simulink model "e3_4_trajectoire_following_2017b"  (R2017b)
settings: Solver=FixedStepAuto  StartTime=0.0  StopTime=150  FixedStep=sampleTime  RelTol=1e-3  EnableMultiTasking=on
InitFcn:
  | start;
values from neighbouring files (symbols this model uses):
  k_d_x = 1.65    [start.m]    (also in StartSimulation.m = 1.5; startSimulation.m = 1.5)
  k_d_y = 1.52    [start.m]    (also in StartSimulation.m = 1.5; startSimulation.m = 1.5)
  k_d_yaw = 1    [start.m]    (also in StartSimulation.m; startSimulation.m)
  k_d_z = 0.5    [start.m]    (also in StartSimulation.m; startSimulation.m)
  k_i_x = 0.9    [start.m]    (also in StartSimulation.m = 0.01; startSimulation.m = 0.01)
  k_i_y = 0.91    [start.m]    (also in StartSimulation.m = 0.01; startSimulation.m = 0.01)
  k_i_yaw = 0.01    [start.m]    (also in StartSimulation.m; startSimulation.m)
  k_i_z = 0.01    [start.m]    (also in StartSimulation.m; startSimulation.m)
  k_p_x = 1.9    [start.m]    (also in StartSimulation.m = 1.2; startSimulation.m = 1.2)
  k_p_y = 1.9    [start.m]    (also in StartSimulation.m = 1.5; startSimulation.m = 1.5)
  k_p_yaw = 2    [start.m]    (also in StartSimulation.m; startSimulation.m)
  k_p_z = 2    [start.m]    (also in StartSimulation.m; startSimulation.m)
  saturation_psi = 2    [start.m]    (also in StartSimulation.m; startSimulation.m)
  saturation_x = 2    [start.m]    (also in StartSimulation.m; startSimulation.m)
  saturation_y = 2    [start.m]    (also in StartSimulation.m; startSimulation.m)
  saturation_z = 2    [start.m]    (also in StartSimulation.m; startSimulation.m)
libraries: simulink x36, aerolibanimutils x1

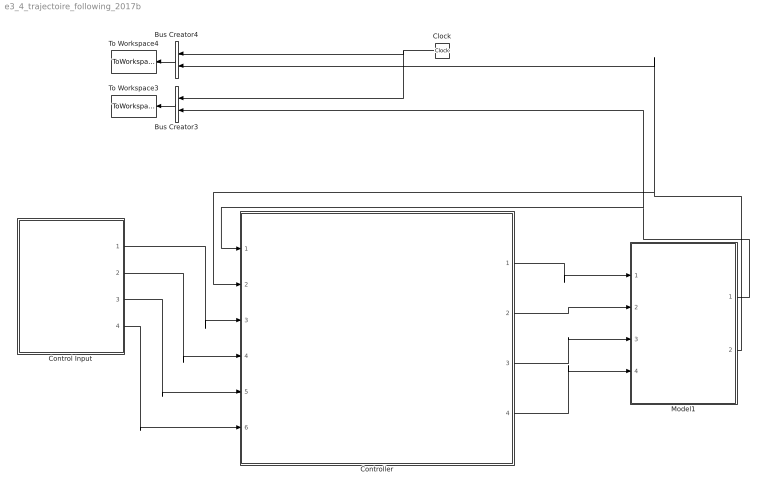
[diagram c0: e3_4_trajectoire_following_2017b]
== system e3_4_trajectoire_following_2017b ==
  Bus Creator3 : BusCreator  Inputs=2
  Bus Creator4 : BusCreator  Inputs=2
  Clock : Clock
  Control Input : Subsystem
  Controller : Subsystem
  Model1 : Subsystem
  To Workspace3 : ToWorkspace  VariableName=r1_pos_array1  SampleTime=-1
  To Workspace4 : ToWorkspace  VariableName=r1_vel_array1  SampleTime=-1
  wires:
  Controller/2(Controller Output Y) -> Model1/2(uy)
  Controller/3(Controller Output H) -> Model1/3(uz)
  Controller/4(Controller Output Psi) -> Model1/4(upsi)
  Model1/2(Output Velocity1) -> Bus Creator4/2, Controller/2(Feedback Velocity)
  Model1/1(Output Postion1) -> Bus Creator3/2, Controller/1(Feedback Position)
  Bus Creator3/1 -> To Workspace3/1
  Clock/1 -> Bus Creator3/1, Bus Creator4/1
  Bus Creator4/1 -> To Workspace4/1
  Control Input/2(uy) -> Controller/4(Control input Y)
  Control Input/1(ux) -> Controller/3(Control input X)
  Control Input/3(uz) -> Controller/5(Control input H)
  Control Input/4(upsi) -> Controller/6(Control input Psi)
  Controller/1(Controller Output X) -> Model1/1(ux)

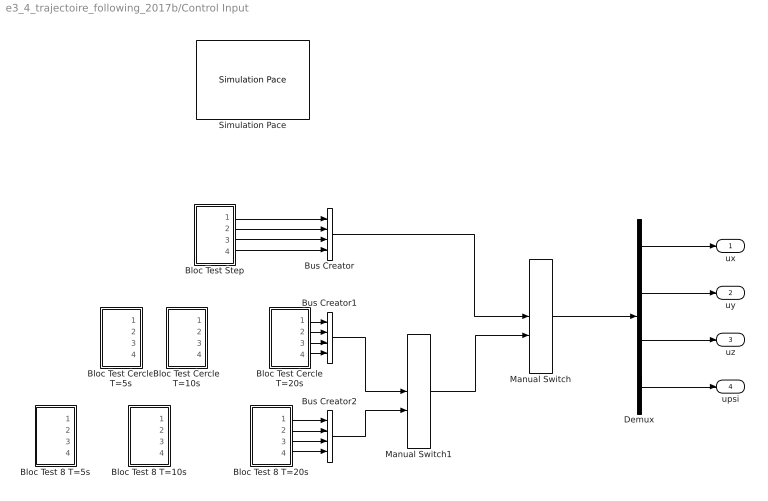
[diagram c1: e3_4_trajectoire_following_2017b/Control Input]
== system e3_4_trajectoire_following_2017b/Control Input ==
  Bloc Test 8 T=10s : Subsystem
  Bloc Test 8 T=20s : Subsystem
  Bloc Test 8 T=5s : Subsystem
  Bloc Test Cercle T=10s : Subsystem
  Bloc Test Cercle T=20s : Subsystem
  Bloc Test Cercle T=5s : Subsystem
  Bloc Test Step : Subsystem
  Bus Creator : BusCreator  Inputs=4
  Bus Creator1 : BusCreator  Inputs=4
  Bus Creator2 : BusCreator  Inputs=4
  Demux : Demux
  Manual Switch : ManualSwitch  CurrentSetting=0
  Manual Switch1 : ManualSwitch
  Simulation Pace : aerolibanimutils/Simulation Pace  SimulationPace=100  SleepMode=MATLAB Thread  OutputPaceError=off  SampleTime=-1
  ux : Outport  VectorParamsAs1DForOutWhenUnconnected=off
  uy : Outport  Port=2  VectorParamsAs1DForOutWhenUnconnected=off
  uz : Outport  Port=3  VectorParamsAs1DForOutWhenUnconnected=off
  upsi : Outport  Port=4  VectorParamsAs1DForOutWhenUnconnected=off
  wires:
  Demux/2 -> uy/1
  Demux/1 -> ux/1
  Bloc Test Step/2(uy) -> Bus Creator/2
  Demux/3 -> uz/1
  Demux/4 -> upsi/1
  Bloc Test Step/4(upsi) -> Bus Creator/4
  Bloc Test Step/3(uz) -> Bus Creator/3
  Bloc Test Step/1(ux) -> Bus Creator/1
  Bus Creator/1 -> Manual Switch/1
  Bus Creator1/1 -> Manual Switch1/1
  Bus Creator2/1 -> Manual Switch1/2
  Manual Switch/1 -> Demux/1
  Manual Switch1/1 -> Manual Switch/2
  Bloc Test 8 T=20s/1(ux) -> Bus Creator2/1
  Bloc Test 8 T=20s/2(uy) -> Bus Creator2/2
  Bloc Test 8 T=20s/3(uz) -> Bus Creator2/3
  Bloc Test 8 T=20s/4(upsi) -> Bus Creator2/4
  Bloc Test Cercle T=20s/1(ux) -> Bus Creator1/1
  Bloc Test Cercle T=20s/2(uy) -> Bus Creator1/2
  Bloc Test Cercle T=20s/3(uz) -> Bus Creator1/3
  Bloc Test Cercle T=20s/4(upsi) -> Bus Creator1/4

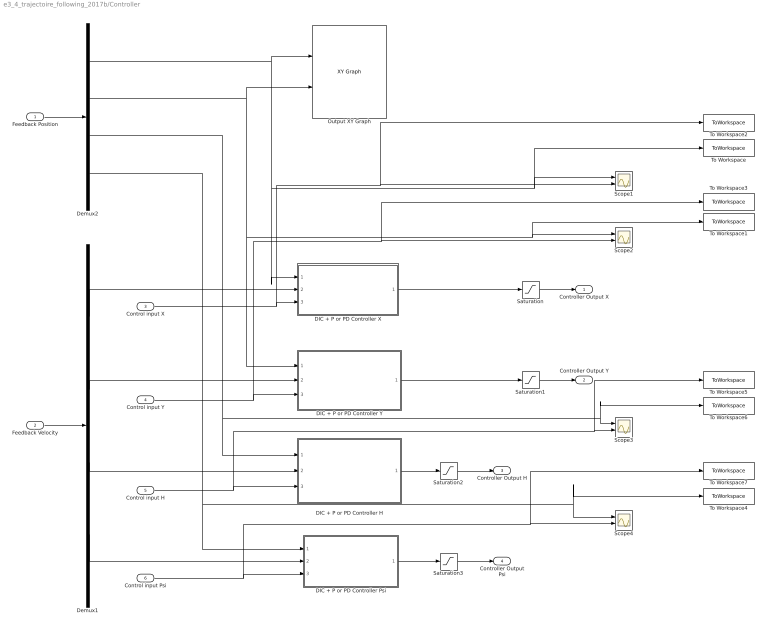
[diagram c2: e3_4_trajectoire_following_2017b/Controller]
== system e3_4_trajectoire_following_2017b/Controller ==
  Feedback Position : Inport
  Feedback Velocity : Inport  Port=2
  Control input X : Inport  Port=3
  Control input Y : Inport  Port=4
  Control input H : Inport  Port=5
  Control input Psi : Inport  Port=6
  DIC + P or PD Controller H : Subsystem
  DIC + P or PD Controller Psi : Subsystem
  DIC + P or PD Controller X : Subsystem
  DIC + P or PD Controller Y : Subsystem
  Demux1 : Demux
  Demux2 : Demux
  Output XY Graph : simulink/Sinks/XY Graph  xmin=-1  xmax=1  ymin=-1  ymax=1  st=-1
  Saturation : Saturate  UpperLimit=saturation_x  LowerLimit=-saturation_x
  Saturation1 : Saturate  UpperLimit=saturation_y  LowerLimit=-saturation_y
  Saturation2 : Saturate  UpperLimit=saturation_z  LowerLimit=-saturation_z
  Saturation3 : Saturate  UpperLimit=saturation_psi  LowerLimit=-saturation_psi
  Scope{1..4} (4 alike) : Scope  NumInputPorts=2
  To Workspace : ToWorkspace  VariableName=N4_Step1_Out_X  SampleTime=-1
  To Workspace1 : ToWorkspace  VariableName=N4_Step1_Out_Y  SampleTime=-1
  To Workspace2 : ToWorkspace  VariableName=N4_Step1_In_X  SampleTime=-1
  To Workspace3 : ToWorkspace  VariableName=N4_Step1_In_Y  SampleTime=-1
  To Workspace4 : ToWorkspace  VariableName=N4_Step1_Out_Psi  SampleTime=-1
  To Workspace5 : ToWorkspace  VariableName=N4_Step1_In_H  SampleTime=-1
  To Workspace6 : ToWorkspace  VariableName=N4_Step1_Out_H  SampleTime=-1
  To Workspace7 : ToWorkspace  VariableName=N4_Step1_In_Psi  SampleTime=-1
  Controller Output X : Outport  VectorParamsAs1DForOutWhenUnconnected=off
  Controller Output Y : Outport  Port=2  VectorParamsAs1DForOutWhenUnconnected=off
  Controller Output H : Outport  Port=3  VectorParamsAs1DForOutWhenUnconnected=off
  Controller Output Psi : Outport  Port=4  VectorParamsAs1DForOutWhenUnconnected=off
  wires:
  Feedback Position/1 -> Demux2/1
  Feedback Velocity/1 -> Demux1/1
  Demux1/2 -> DIC + P or PD Controller Y/2(Feedback Velocity Y)
  Demux2/3 -> Scope3/1, To Workspace6/1, DIC + P or PD Controller H/1(Feedback Position H)
  Demux1/1 -> DIC + P or PD Controller X/2(Feedback Velocity X)
  Demux1/3 -> DIC + P or PD Controller H/2(Feedback Velocity H)
  Control input X/1 -> To Workspace2/1, Scope1/2, DIC + P or PD Controller X/3(Control Input X)
  Control input H/1 -> Scope3/2, To Workspace5/1, DIC + P or PD Controller H/3(Control Input H)
  Saturation/1 -> Controller Output X/1
  Saturation1/1 -> Controller Output Y/1
  Saturation2/1 -> Controller Output H/1
  Saturation3/1 -> Controller Output Psi/1
  Control input Y/1 -> Scope2/2, To Workspace3/1, DIC + P or PD Controller Y/3(Control Input Y)
  DIC + P or PD Controller H/1(Controller Output H) -> Saturation2/1
  DIC + P or PD Controller Psi/1(Controller Output Psi) -> Saturation3/1
  Demux2/1 -> DIC + P or PD Controller X/1(Feedback Position X), To Workspace/1, Scope1/1, Output XY Graph/1
  Demux2/2 -> Scope2/1, To Workspace1/1, DIC + P or PD Controller Y/1(Feedback Position Y), Output XY Graph/2
  Demux2/4 -> Scope4/1, To Workspace4/1, DIC + P or PD Controller Psi/1(Feedback Position Psi)
  Demux1/4 -> DIC + P or PD Controller Psi/2(Feedback Velocity Psi)
  Control input Psi/1 -> Scope4/2, To Workspace7/1, DIC + P or PD Controller Psi/3(Control input Psi)
  DIC + P or PD Controller Y/1(Controller Output Y) -> Saturation1/1
  DIC + P or PD Controller X/1(Controller Output X) -> Saturation/1

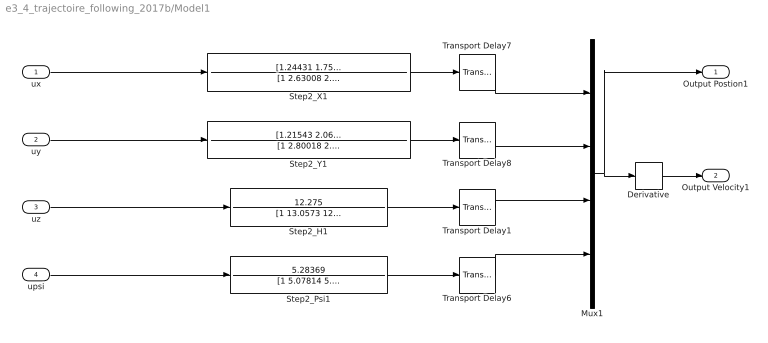
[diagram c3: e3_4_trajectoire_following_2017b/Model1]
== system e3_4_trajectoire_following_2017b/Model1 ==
  ux : Inport
  uy : Inport  Port=2
  uz : Inport  Port=3
  upsi : Inport  Port=4
  Derivative : Derivative
  Mux1 : Mux
  Step2_H1 : TransferFcn  Numerator=12.275  Denominator=[1 13.0573 12.3932]
  Step2_Psi1 : TransferFcn  Numerator=5.28369  Denominator=[1 5.07814 5.37552]
  Step2_X1 : TransferFcn  Numerator=[1.24431 1.75269]  Denominator=[1 2.63008 2.37405 1.95897]
  Step2_Y1 : TransferFcn  Numerator=[1.21543 2.06629]  Denominator=[1 2.80018 2.54762 2.23605]
  Transport Delay1 : TransportDelay  DelayTime=0.0271
  Transport Delay6 : TransportDelay  DelayTime=0.0281
  Transport Delay7 : TransportDelay  DelayTime=0.3778
  Transport Delay8 : TransportDelay  DelayTime=0.3715
  Output Postion1 : Outport
  Output Velocity1 : Outport  Port=2
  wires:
  upsi/1 -> Step2_Psi1/1
  Transport Delay8/1 -> Mux1/2
  Step2_Y1/1 -> Transport Delay8/1
  Step2_Psi1/1 -> Transport Delay6/1
  Transport Delay6/1 -> Mux1/4
  Transport Delay1/1 -> Mux1/3
  ux/1 -> Step2_X1/1
  Step2_X1/1 -> Transport Delay7/1
  Transport Delay7/1 -> Mux1/1
  Step2_H1/1 -> Transport Delay1/1
  uz/1 -> Step2_H1/1
  uy/1 -> Step2_Y1/1
  Derivative/1 -> Output Velocity1/1
  Mux1/1 -> Derivative/1, Output Postion1/1

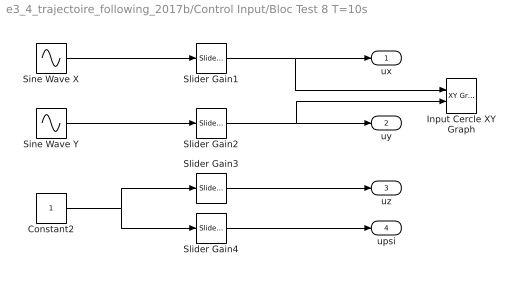
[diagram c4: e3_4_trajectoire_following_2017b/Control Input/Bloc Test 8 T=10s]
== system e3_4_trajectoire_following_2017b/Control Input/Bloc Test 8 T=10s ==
  Constant2 : Constant
  Input Cercle XY Graph : simulink/Sinks/XY Graph  xmin=-1  xmax=1  ymin=-1  ymax=1  st=-1
  Sine Wave X : Sin  Frequency=0.65  SampleTime=0
  Sine Wave Y : Sin  Frequency=1.3  SampleTime=0
  Slider Gain1 : simulink/Math Operations/Slider Gain  gain=1  low=-10  high=10
  Slider Gain2 : simulink/Math Operations/Slider Gain  gain=1  low=-10  high=10
  Slider Gain3 : simulink/Math Operations/Slider Gain  gain=1  low=-3  high=3
  Slider Gain4 : simulink/Math Operations/Slider Gain  gain=0  low=-2  high=2
  ux : Outport  VectorParamsAs1DForOutWhenUnconnected=off
  uy : Outport  Port=2  VectorParamsAs1DForOutWhenUnconnected=off
  uz : Outport  Port=3  VectorParamsAs1DForOutWhenUnconnected=off
  upsi : Outport  Port=4  VectorParamsAs1DForOutWhenUnconnected=off
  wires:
  Slider Gain2/1 -> Input Cercle XY Graph/2, uy/1
  Slider Gain3/1 -> uz/1
  Slider Gain4/1 -> upsi/1
  Slider Gain1/1 -> Input Cercle XY Graph/1, ux/1
  Constant2/1 -> Slider Gain4/1, Slider Gain3/1
  Sine Wave Y/1 -> Slider Gain2/1
  Sine Wave X/1 -> Slider Gain1/1

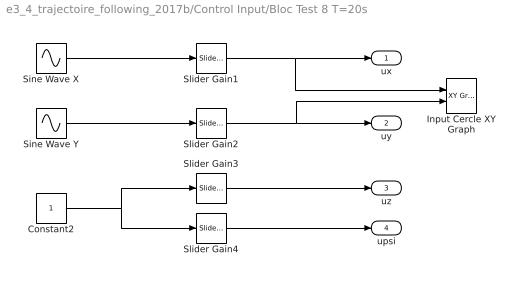
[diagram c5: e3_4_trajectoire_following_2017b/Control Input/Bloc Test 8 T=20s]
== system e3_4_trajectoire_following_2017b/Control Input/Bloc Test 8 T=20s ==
  Constant2 : Constant
  Input Cercle XY Graph : simulink/Sinks/XY Graph  xmin=-1  xmax=1  ymin=-1  ymax=1  st=-1
  Sine Wave X : Sin  Frequency=0.35  SampleTime=0
  Sine Wave Y : Sin  Frequency=0.7  SampleTime=0
  Slider Gain1 : simulink/Math Operations/Slider Gain  gain=1  low=-10  high=10
  Slider Gain2 : simulink/Math Operations/Slider Gain  gain=1  low=-10  high=10
  Slider Gain3 : simulink/Math Operations/Slider Gain  gain=1  low=-3  high=3
  Slider Gain4 : simulink/Math Operations/Slider Gain  gain=0  low=-2  high=2
  ux : Outport  VectorParamsAs1DForOutWhenUnconnected=off
  uy : Outport  Port=2  VectorParamsAs1DForOutWhenUnconnected=off
  uz : Outport  Port=3  VectorParamsAs1DForOutWhenUnconnected=off
  upsi : Outport  Port=4  VectorParamsAs1DForOutWhenUnconnected=off
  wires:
  Slider Gain2/1 -> Input Cercle XY Graph/2, uy/1
  Slider Gain3/1 -> uz/1
  Slider Gain4/1 -> upsi/1
  Slider Gain1/1 -> Input Cercle XY Graph/1, ux/1
  Constant2/1 -> Slider Gain4/1, Slider Gain3/1
  Sine Wave Y/1 -> Slider Gain2/1
  Sine Wave X/1 -> Slider Gain1/1

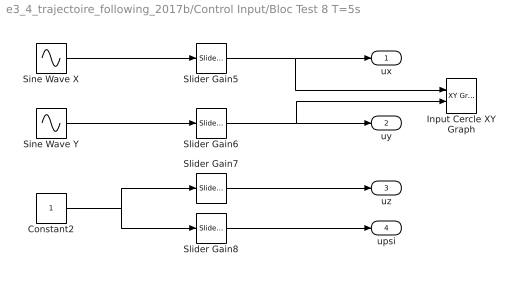
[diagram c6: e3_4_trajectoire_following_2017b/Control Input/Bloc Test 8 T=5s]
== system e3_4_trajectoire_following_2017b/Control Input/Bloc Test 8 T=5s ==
  Constant2 : Constant
  Input Cercle XY Graph : simulink/Sinks/XY Graph  xmin=-1  xmax=1  ymin=-1  ymax=1  st=-1
  Sine Wave X : Sin  SampleTime=0
  Sine Wave Y : Sin  Frequency=2  SampleTime=0
  Slider Gain5 : simulink/Math Operations/Slider Gain  gain=1  low=-10  high=10
  Slider Gain6 : simulink/Math Operations/Slider Gain  gain=1  low=-10  high=10
  Slider Gain7 : simulink/Math Operations/Slider Gain  gain=1  low=-3  high=3
  Slider Gain8 : simulink/Math Operations/Slider Gain  gain=0  low=-2  high=2
  ux : Outport  VectorParamsAs1DForOutWhenUnconnected=off
  uy : Outport  Port=2  VectorParamsAs1DForOutWhenUnconnected=off
  uz : Outport  Port=3  VectorParamsAs1DForOutWhenUnconnected=off
  upsi : Outport  Port=4  VectorParamsAs1DForOutWhenUnconnected=off
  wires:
  Slider Gain6/1 -> Input Cercle XY Graph/2, uy/1
  Slider Gain7/1 -> uz/1
  Slider Gain8/1 -> upsi/1
  Slider Gain5/1 -> Input Cercle XY Graph/1, ux/1
  Constant2/1 -> Slider Gain8/1, Slider Gain7/1
  Sine Wave Y/1 -> Slider Gain6/1
  Sine Wave X/1 -> Slider Gain5/1

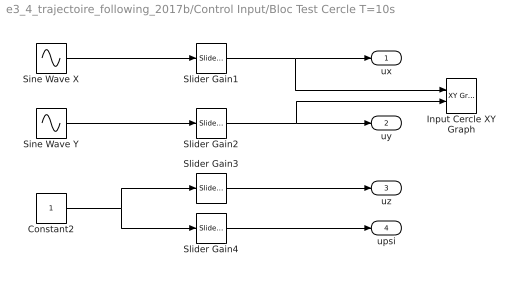
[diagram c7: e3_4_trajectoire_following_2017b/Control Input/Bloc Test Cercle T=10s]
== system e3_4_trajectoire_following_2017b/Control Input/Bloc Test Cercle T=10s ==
  Constant2 : Constant
  Input Cercle XY Graph : simulink/Sinks/XY Graph  xmin=-1  xmax=1  ymin=-1  ymax=1  st=-1
  Sine Wave X : Sin  Frequency=0.65  SampleTime=0
  Sine Wave Y : Sin  Frequency=0.65  Phase=pi/2  SampleTime=0
  Slider Gain1 : simulink/Math Operations/Slider Gain  gain=1  low=-10  high=10
  Slider Gain2 : simulink/Math Operations/Slider Gain  gain=1  low=-10  high=10
  Slider Gain3 : simulink/Math Operations/Slider Gain  gain=1  low=-3  high=3
  Slider Gain4 : simulink/Math Operations/Slider Gain  gain=0  low=-2  high=2
  ux : Outport  VectorParamsAs1DForOutWhenUnconnected=off
  uy : Outport  Port=2  VectorParamsAs1DForOutWhenUnconnected=off
  uz : Outport  Port=3  VectorParamsAs1DForOutWhenUnconnected=off
  upsi : Outport  Port=4  VectorParamsAs1DForOutWhenUnconnected=off
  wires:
  Slider Gain2/1 -> Input Cercle XY Graph/2, uy/1
  Slider Gain3/1 -> uz/1
  Slider Gain4/1 -> upsi/1
  Slider Gain1/1 -> Input Cercle XY Graph/1, ux/1
  Constant2/1 -> Slider Gain4/1, Slider Gain3/1
  Sine Wave Y/1 -> Slider Gain2/1
  Sine Wave X/1 -> Slider Gain1/1

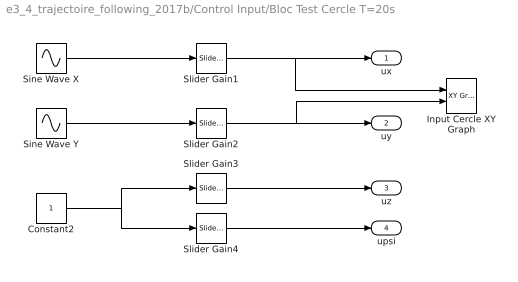
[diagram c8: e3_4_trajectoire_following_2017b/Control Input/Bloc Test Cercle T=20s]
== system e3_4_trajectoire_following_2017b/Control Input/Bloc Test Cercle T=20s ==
  Constant2 : Constant
  Input Cercle XY Graph : simulink/Sinks/XY Graph  xmin=-1  xmax=1  ymin=-1  ymax=1  st=-1
  Sine Wave X : Sin  Frequency=0.35  SampleTime=0
  Sine Wave Y : Sin  Frequency=0.35  Phase=pi/2  SampleTime=0
  Slider Gain1 : simulink/Math Operations/Slider Gain  gain=1  low=-10  high=10
  Slider Gain2 : simulink/Math Operations/Slider Gain  gain=1  low=-10  high=10
  Slider Gain3 : simulink/Math Operations/Slider Gain  gain=1  low=-3  high=3
  Slider Gain4 : simulink/Math Operations/Slider Gain  gain=0  low=-2  high=2
  ux : Outport  VectorParamsAs1DForOutWhenUnconnected=off
  uy : Outport  Port=2  VectorParamsAs1DForOutWhenUnconnected=off
  uz : Outport  Port=3  VectorParamsAs1DForOutWhenUnconnected=off
  upsi : Outport  Port=4  VectorParamsAs1DForOutWhenUnconnected=off
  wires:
  Slider Gain2/1 -> Input Cercle XY Graph/2, uy/1
  Slider Gain3/1 -> uz/1
  Slider Gain4/1 -> upsi/1
  Slider Gain1/1 -> Input Cercle XY Graph/1, ux/1
  Constant2/1 -> Slider Gain4/1, Slider Gain3/1
  Sine Wave Y/1 -> Slider Gain2/1
  Sine Wave X/1 -> Slider Gain1/1

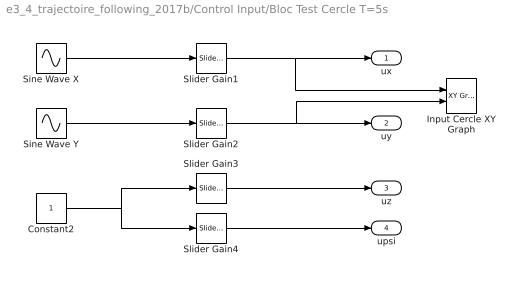
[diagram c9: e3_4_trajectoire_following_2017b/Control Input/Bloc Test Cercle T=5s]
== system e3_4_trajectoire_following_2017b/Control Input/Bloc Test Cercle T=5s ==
  Constant2 : Constant
  Input Cercle XY Graph : simulink/Sinks/XY Graph  xmin=-1  xmax=1  ymin=-1  ymax=1  st=-1
  Sine Wave X : Sin  SampleTime=0
  Sine Wave Y : Sin  Phase=pi/2  SampleTime=0
  Slider Gain1 : simulink/Math Operations/Slider Gain  gain=1  low=-10  high=10
  Slider Gain2 : simulink/Math Operations/Slider Gain  gain=1  low=-10  high=10
  Slider Gain3 : simulink/Math Operations/Slider Gain  gain=1  low=-3  high=3
  Slider Gain4 : simulink/Math Operations/Slider Gain  gain=0  low=-2  high=2
  ux : Outport  VectorParamsAs1DForOutWhenUnconnected=off
  uy : Outport  Port=2  VectorParamsAs1DForOutWhenUnconnected=off
  uz : Outport  Port=3  VectorParamsAs1DForOutWhenUnconnected=off
  upsi : Outport  Port=4  VectorParamsAs1DForOutWhenUnconnected=off
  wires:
  Slider Gain2/1 -> Input Cercle XY Graph/2, uy/1
  Slider Gain3/1 -> uz/1
  Slider Gain4/1 -> upsi/1
  Slider Gain1/1 -> Input Cercle XY Graph/1, ux/1
  Constant2/1 -> Slider Gain4/1, Slider Gain3/1
  Sine Wave Y/1 -> Slider Gain2/1
  Sine Wave X/1 -> Slider Gain1/1

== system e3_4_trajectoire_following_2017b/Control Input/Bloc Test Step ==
  Constant2 : Constant
  Input Segment XY Graph : simulink/Sinks/XY Graph  xmin=-1  xmax=1  ymin=-1  ymax=1  st=-1
  Slider Gain1 : simulink/Math Operations/Slider Gain  gain=1  low=-10  high=10
  Slider Gain2 : simulink/Math Operations/Slider Gain  gain=1  low=-10  high=10
  Slider Gain3 : simulink/Math Operations/Slider Gain  gain=1  low=-2  high=2
  Slider Gain4 : simulink/Math Operations/Slider Gain  gain=0  low=-2  high=2
  Step X1 : Step  Time=5  SampleTime=0
  ux : Outport  VectorParamsAs1DForOutWhenUnconnected=off
  uy : Outport  Port=2  VectorParamsAs1DForOutWhenUnconnected=off
  uz : Outport  Port=3  VectorParamsAs1DForOutWhenUnconnected=off
  upsi : Outport  Port=4  VectorParamsAs1DForOutWhenUnconnected=off
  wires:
  Slider Gain1/1 -> Input Segment XY Graph/1, ux/1
  Slider Gain2/1 -> Input Segment XY Graph/2, uy/1
  Slider Gain3/1 -> uz/1
  Slider Gain4/1 -> upsi/1
  Step X1/1 -> Slider Gain3/1, Slider Gain4/1, Slider Gain2/1, Slider Gain1/1

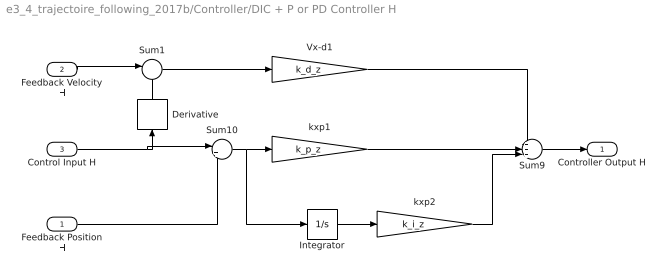
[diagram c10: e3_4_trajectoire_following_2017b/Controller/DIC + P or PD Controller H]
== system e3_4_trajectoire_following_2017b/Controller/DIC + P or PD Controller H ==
  Feedback Position H : Inport
  Feedback Velocity H : Inport  Port=2
  Control Input H : Inport  Port=3
  Derivative : Derivative
  Integrator : Integrator
  Sum1 : Sum  Inputs=|-+
  Sum10 : Sum  Inputs=|+-
  Sum9 : Sum  Inputs=+++|
  Vx-d1 : Gain  Gain=k_d_z
  kxp1 : Gain  Gain=k_p_z
  kxp2 : Gain  Gain=k_i_z
  Controller Output H : Outport  VectorParamsAs1DForOutWhenUnconnected=off
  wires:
  Sum9/1 -> Controller Output H/1
  Sum10/1 -> Integrator/1, kxp1/1
  kxp1/1 -> Sum9/2
  Vx-d1/1 -> Sum9/1
  Feedback Velocity H/1 -> Sum1/1
  Sum1/1 -> Vx-d1/1
  Integrator/1 -> kxp2/1
  kxp2/1 -> Sum9/3
  Control Input H/1 -> Sum10/1, Derivative/1
  Feedback Position H/1 -> Sum10/2
  Derivative/1 -> Sum1/2

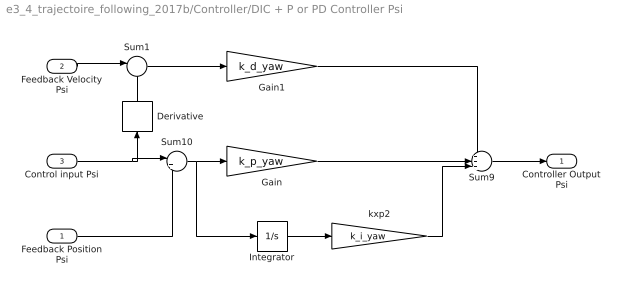
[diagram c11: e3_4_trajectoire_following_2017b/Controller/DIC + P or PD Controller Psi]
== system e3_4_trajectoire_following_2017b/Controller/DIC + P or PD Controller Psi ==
  Feedback Position Psi : Inport
  Feedback Velocity Psi : Inport  Port=2
  Control input Psi : Inport  Port=3
  Derivative : Derivative
  Gain : Gain  Gain=k_p_yaw
  Gain1 : Gain  Gain=k_d_yaw
  Integrator : Integrator
  Sum1 : Sum  Inputs=|-+
  Sum10 : Sum  Inputs=|+-
  Sum9 : Sum  Inputs=+++|
  kxp2 : Gain  Gain=k_i_yaw
  Controller Output Psi : Outport  VectorParamsAs1DForOutWhenUnconnected=off
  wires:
  Sum9/1 -> Controller Output Psi/1
  kxp2/1 -> Sum9/3
  Control input Psi/1 -> Sum10/1, Derivative/1
  Gain1/1 -> Sum9/1
  Sum10/1 -> Gain/1, Integrator/1
  Integrator/1 -> kxp2/1
  Feedback Velocity Psi/1 -> Sum1/1
  Sum1/1 -> Gain1/1
  Gain/1 -> Sum9/2
  Derivative/1 -> Sum1/2
  Feedback Position Psi/1 -> Sum10/2

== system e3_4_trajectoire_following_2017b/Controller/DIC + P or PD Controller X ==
  Feedback Position X : Inport
  Feedback Velocity X : Inport  Port=2
  Control Input X : Inport  Port=3
  Derivative : Derivative
  Integrator : Integrator
  Sum1 : Sum  Inputs=|-+
  Sum10 : Sum  Inputs=|+-
  Sum9 : Sum  Inputs=+++|
  Vx-d3 : Gain  Gain=k_d_x
  kxp2 : Gain  Gain=k_i_x
  kxp3 : Gain  Gain=k_p_x
  Controller Output X : Outport  VectorParamsAs1DForOutWhenUnconnected=off
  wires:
  Sum9/1 -> Controller Output X/1
  Feedback Velocity X/1 -> Sum1/1
  Feedback Position X/1 -> Sum10/2
  Sum1/1 -> Vx-d3/1
  Integrator/1 -> kxp2/1
  kxp3/1 -> Sum9/2
  Vx-d3/1 -> Sum9/1
  Sum10/1 -> kxp3/1, Integrator/1
  Derivative/1 -> Sum1/2
  kxp2/1 -> Sum9/3
  Control Input X/1 -> Sum10/1, Derivative/1

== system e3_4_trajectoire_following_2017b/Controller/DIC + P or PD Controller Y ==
  Feedback Position Y : Inport
  Feedback Velocity Y : Inport  Port=2
  Control Input Y : Inport  Port=3
  Derivative : Derivative
  Integrator : Integrator
  Sum1 : Sum  Inputs=|-+
  Sum10 : Sum  Inputs=|+-
  Sum9 : Sum  Inputs=+++|
  Vx-d3 : Gain  Gain=k_d_y
  kxp2 : Gain  Gain=k_i_y
  kxp3 : Gain  Gain=k_p_y
  Controller Output Y : Outport  VectorParamsAs1DForOutWhenUnconnected=off
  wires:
  Feedback Position Y/1 -> Sum10/2
  Control Input Y/1 -> Sum10/1, Derivative/1
  Sum9/1 -> Controller Output Y/1
  Integrator/1 -> kxp2/1
  kxp3/1 -> Sum9/2
  Sum10/1 -> kxp3/1, Integrator/1
  kxp2/1 -> Sum9/3
  Vx-d3/1 -> Sum9/1
  Feedback Velocity Y/1 -> Sum1/1
  Sum1/1 -> Vx-d3/1
  Derivative/1 -> Sum1/2
